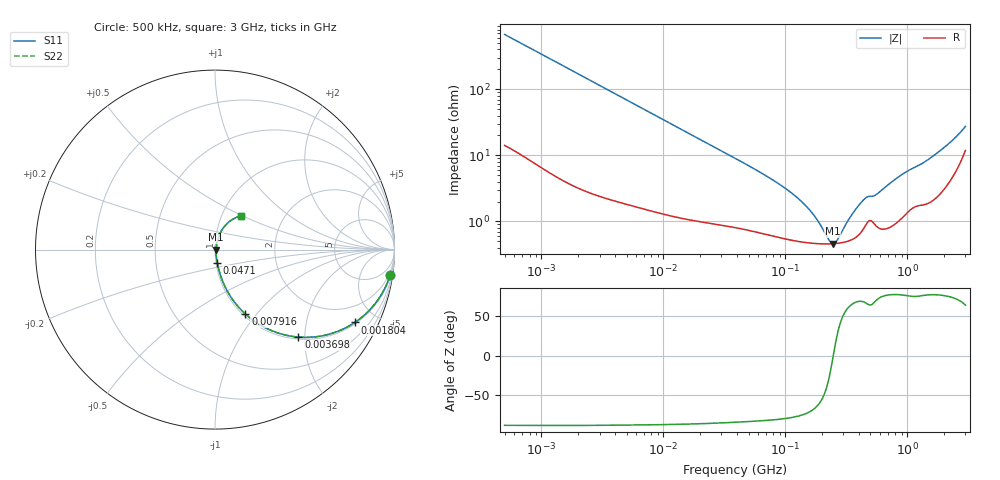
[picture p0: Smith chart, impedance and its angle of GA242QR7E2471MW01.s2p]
!Murata Part Number: GA242QR7E2471MW01
!These Parameters are Measured in Series Mode Connection
!Data Generated on Jun 19, 2026
!  o--ll--o
!Port1  Port2
!  o------o
!Operation Temp=25[degC], DC Bias Voltage=0[V]
!Freq. Start=500[kHz] Stop=3[GHz] 401[Steps]
# Hz S RI R 50
!Freq.(Hz) S11(Real) S11(Imag) S21(Real) S21(Imag) S12(Real) S12(Imag) S22(Real) S22(Imag)
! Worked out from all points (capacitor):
!   401 points, 500 kHz to 3 GHz, reference 50 ohm
!   read as one part in series: C = 470 pF near 522.2 kHz
!   lowest |Z| = 461 mohm at 246 MHz (marker M1)
!   series resonance near 247.7 MHz, so ESL is about 880 pH
!   S11 on the Smith chart (normalised r, x): 500 kHz: 1, -13; 1.804 MHz: 1.07, -3.80; 3.698 MHz: 1.04, -1.86; 7.916 MHz: 1.03, -0.88; 47.1 MHz: 1.02, -0.15; 3 GHz: 1.24, +0.49
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500000  0.9756 -0.1441  0.0244 0.1441  0.0244 0.1441  0.9756 -0.1441
1024867  0.9128 -0.2728  0.0872 0.2728  0.0872 0.2728  0.9128 -0.2728
1804045  0.7785 -0.4062  0.2215 0.4062  0.2215 0.4062  0.7785 -0.4062
2146893  0.7146 -0.4422  0.2854 0.4422  0.2854 0.4422  0.7146 -0.4422
3697812  0.465 -0.4875  0.535 0.4875  0.535 0.4875  0.465 -0.4875
7916497  0.1692 -0.3588  0.8308 0.3588  0.8308 0.3588  0.1692 -0.3588
9218297  0.1331 -0.3224  0.8669 0.3224  0.8669 0.3224  0.1331 -0.3224
1.658349e7  0.0516 -0.1976  0.9484 0.1976  0.9484 0.1976  0.0516 -0.1976
3.958139e7  0.0155 -0.0863  0.9845 0.0863  0.9845 0.0863  0.0155 -0.0863
4.710359e7  0.0128 -0.0724  0.9872 0.0724  0.9872 0.0724  0.0128 -0.0724
1.030594e8  0.00623 -0.0297  0.9938 0.0297  0.9938 0.0297  0.00623 -0.0297
1.337926e8  0.00529 -0.0198  0.9947 0.0198  0.9947 0.0198  0.00529 -0.0198
1.662976e8  0.00481 -0.0125  0.9952 0.0125  0.9952 0.0125  0.00481 -0.0125
2.304447e8  0.00456 -0.00223  0.9954 0.00223  0.9954 0.00223  0.00456 -0.00223
2.459817e8  0.00458 -0.000213  0.9954 0.000213  0.9954 0.000213  0.00458 -0.000213
2.683393e8  0.00465 0.0025  0.9953 -0.0025  0.9953 -0.0025  0.00465 0.0025
3.408658e8  0.00525 0.0103  0.9948 -0.0103  0.9948 -0.0103  0.00525 0.0103
4.329947e8  0.00779 0.019  0.9922 -0.019  0.9922 -0.019  0.00779 0.019
5.500242e8  0.00921 0.0231  0.9908 -0.0231  0.9908 -0.0231  0.00921 0.0231
7.140462e8  0.00929 0.0357  0.9907 -0.0357  0.9907 -0.0357  0.00929 0.0357
1.941841e9  0.0411 0.1135  0.9589 -0.1135  0.9589 -0.1135  0.0411 0.1135
3e9  0.1475 0.1882  0.8525 -0.1882  0.8525 -0.1882  0.1475 0.1882
